[IBIS Ver]   4.1
[File Name]   rm57l843zwt.ibs
[File Rev]   1.0
[Date]   Mon Sep 1 2015 15:18:58
[Source]   Texas Instruments, Inc.
[Notes]   Revision History:
   1.0: initial release
   THE CONTENTS ARE SUBJECT TO CHANGE
   WITHOUT PRIOR NOTICE,IF NECESSARY.
[Disclaimer] Please be aware that in the absence of a written agreement
   Texas Instruments(TI) assumes no liability for:
   (1) The accuracy of the IBIS models provided to your company
   (2) The proper functioning of these Models in your design
   or for any resulting applications;or
   (3) Infringement of patents,copyrights or intellectual
   property rights resulting from your use of these models.
   TI provides IBIS Models as a service to our customers and
   therefore reserves the right to limit distribution of the
   Models.
[Copyright]   Property of Texas Instruments Incorporated.
   Unauthorised reproduction and/or distribution is strictly.
   prohibited.
   This product is protected under copyright law and trade
   secret law as an unpublished work.
   Created 2015,(C) Copyright 2015
   Texas Instruments Incorporated., All Rights Reserved.
   These commodities are under the U.S. Government
   distribution license control.As such,they are not to be
   re-exported without the prior approval of the
   U.S. Department of Commerce.
[Component]   rm57l843zwt
[Manufacturer]   Texas Instruments
[Package]
|variable   typ   min   max
R_pkg   167.768m   72.6527m   328.833m
L_pkg   2.60458nH   0.744426nH   6.40059nH
C_pkg   0.769905pF   0.48274pF   1.90756pF
[Pin] signal_name   model_name   R_pin   L_pin   C_pin
N19   AD1EVT/MII_RX_ER/RMII_RX_ER/NTZ1_1   BQ0210FS_PD_3X2_7LM_N19   180.1m   2.91nH   0.5019pF
T10   AD2EVT   BQ0210FS_PD_3X2_7LM_T10   191.2m   3.039nH  0.6641pF
B10   DCAN1RX   BQ0210FS_PU_3X2_7LM_B10   168.1m   2.756nH  0.712pF
A10   DCAN1TX   BQ0210FS_PU_3X2_7LM_A10   2190m   3.509nH  0.6666pF
H1   DCAN2RX   BQ0210FS_PU_3X2_7LM_H1   209.7m   3.041nH  0.5571pF
H2   DCAN2TX   BQ0210FS_PU_3X2_7LM_H2   161.2m   2.424nH  0.6686pF
M19   DCAN3RX   BQ0210FS_PU_3X2_7LM_M19   212.9m   3.153nH  0.5852pF
M18   DCAN3TX   BQ0210FS_PU_3X2_7LM_M18   195.7m   2.562nH  0.584pF
F17   DMM_CLK   BQ0210FS_PU_3X2_7LM_F17   159.7m   2.313nH  0.8981pF
L19   DMM_DATA[0]   BQ0210FS_PU_3X2_7LM_L19   211.2m   3.159nH  0.62pF
L18   DMM_DATA[1]   BQ0210FS_PU_3X2_7LM_L18   198.1m   2.749nH  0.6265pF
F16   DMM_NENA   BQ0210FS_PU_3X2_7LM_F16   1790m   2.494nH  1.017pF
J16   DMM_SYNC   BQ0210FS_PU_3X2_7LM_J16   153.5m   1.923nH  0.7789pF
A12   ECLK1   BQ0215FS_PD_3X2_V2_7LM_A12   227.3m   3.717nH  0.7204pF
D4   EMIF_ADDR[0]/N2HET2[1]   BQ0215FS_PD_3X2_7LM_D4   1070m   1.533nH  0.7807pF
C8   EMIF_ADDR[10]/RTP_DATA[9]   BQ0212FS_PD_3X2_7LM_C8   188.2m   2.407nH  0.6629pF
C9   EMIF_ADDR[11]/RTP_DATA[8]   BQ0212FS_PD_3X2_7LM_C9   202.5m   2.785nH  0.7576pF
C10   EMIF_ADDR[12]/RTP_DATA[6]   BQ0212FS_PD_3X2_7LM_C10   111.1m   1.862nH  0.7207pF
C11   EMIF_ADDR[13]/RTP_DATA[5]   BQ0212FS_PD_3X2_7LM_C11   142.7m   2.016nH  0.7216pF
C12   EMIF_ADDR[14]/RTP_DATA[4]   BQ0212FS_PD_3X2_7LM_C12   1920m   2.49nH   0.665pF
C13   EMIF_ADDR[15]/RTP_DATA[3]   BQ0212FS_PD_3X2_7LM_C13   148.4m   2.075nH  0.7037pF
D14   EMIF_ADDR[16]/RTP_DATA[2]   BQ0212FS_PD_3X2_7LM_D14   214.4m   2.798nH  0.7339pF
C14   EMIF_ADDR[17]/RTP_DATA[1]   BQ0212FS_PD_3X2_7LM_C14   133.3m   1.757nH  0.6447pF
D15   EMIF_ADDR[18]/RTP_DATA[0]   BQ0212FS_PD_3X2_7LM_D15   88.7m   1.066nH  0.6122pF
C15   EMIF_ADDR[19]/RTP_NENA   BQ0212FS_PU_3X2_7LM_C15   98.16m   1.386nH  0.6734pF
D5   EMIF_ADDR[1]/N2HET2[3]   BQ0215FS_PD_3X2_7LM_D5   155.7m   2.37nH   0.7927pF
C16   EMIF_ADDR[20]/RTP_NSYNC   BQ0212FS_PU_3X2_7LM_C16   126.9m   2.354nH  0.7879pF
C17   EMIF_ADDR[21]/RTP_CLK   BQ0212FS_PD_3X2_7LM_C17   179.7m   3.038nH  0.9204pF
C4   EMIF_ADDR[6]/RTP_DATA[13]/N2HET2[11]   BQ0215FS_PD_3X2_7LM_C4   217.2m   3.345nH  0.7595pF
C5   EMIF_ADDR[7]/RTP_DATA[12]/N2HET2[13]   BQ0215FS_PD_3X2_7LM_C5   209.2m   3.071nH  0.7332pF
C6   EMIF_ADDR[8]/RTP_DATA[11]/N2HET2[15]   BQ0215FS_PD_3X2_7LM_C6   151.8m   2.305nH  0.7583pF
C7   EMIF_ADDR[9]/RTP_DATA[10]   BQ0212FS_PD_3X2_7LM_C7   2130m   3.027nH  0.7353pF
D16   EMIF_BA[1]/N2HET2[5]   BQ0215FS_PD_3X2_7LM_D16   103.4m   1.556nH  0.6773pF
L3   EMIF_CKE   BQ0212FS_3X2_7LM_L3   188.4m   2.315nH  0.6502pF
R4   EMIF_NCAS/GIOB[3]   BQ0215FS_PD_3X2_7LM_R4   98.03m   1.629nH  0.901pF
N17   EMIF_NCS[0]/RTP_DATA[15]/N2HET2[7]   BQ0215FS_PD_3X2_7LM_N17   215.8m   2.667nH  0.6805pF
L17   EMIF_NCS[2]/GIOB[4]   BQ0215FS_PD_3X2_7LM_L17   1930m   2.377nH  0.6608pF
K17   EMIF_NCS[3]/RTP_DATA[14]/N2HET2[9]   BQ0215FS_PD_3X2_7LM_K17   140.2m   1.913nH  0.6591pF
M17   EMIF_NCS[4]/RTP_DATA[7]/GIOB[5]   BQ0215FS_PD_3X2_7LM_M17   141.2m   1.851nH  0.622pF
R3   EMIF_NRAS/GIOB[6]   BQ0215FS_PD_3X2_7LM_R3   169.2m   2.599nH  0.9236pF
P3   EMIF_NWAIT/GIOB[7]   BQ0210FS_PU_3X2_7LM_P3   225.8m   3.417nH  0.7552pF
D17   EMIF_NWE/EMIF_RNW   BQ0212FS_3X2_7LM_D17   248.5m   4.299nH  0.9019pF
D9   EPWM1A   BQ0212FS_3X2_7LM_D9   154.3m   2.317nH  0.7824pF
D10   EPWM1B   BQ0212FS_3X2_7LM_D10   157.6m   2.386nH  0.7576pF
R12   ETMDATA[0]   BQ0212FS_PD_3X2_7LM_R12   202.1m   3.095nH  1.034pF
E7   ETMDATA[10]/EMIF_ADDR[3]   BQ0212FS_PD_3X2_7LM_E7   155.1m   2.109nH  0.8648pF
E6   ETMDATA[11]/EMIF_ADDR[2]   BQ0212FS_PD_3X2_7LM_E6   152.7m   2.049nH  0.8297pF
E13   ETMDATA[12]/EMIF_BA[0]   BQ0212FS_PD_3X2_7LM_E13   150.6m   1.764nH  0.8299pF
E12   ETMDATA[13]/EMIF_NOE   BQ0212FS_PD_3X2_7LM_E12   84.46m   0.9329nH 0.7552pF
E11   ETMDATA[14]/EMIF_NDQM[1]   BQ0212FS_PD_3X2_7LM_E11   153.2m   2.043nH  0.8118pF
E10   ETMDATA[15]/EMIF_NDQM[0]   BQ0212FS_PD_3X2_7LM_E10   109.9m   1.609nH  0.8404pF
K15   ETMDATA[16]/EMIF_DATA[0]   BQ0212FS_PD_3X2_7LM_K15   159.5m   1.94nH   0.8165pF
L15   ETMDATA[17]/EMIF_DATA[1]   BQ0212FS_PD_3X2_7LM_L15   84.09m   0.8806nH 0.7489pF
M15   ETMDATA[18]/EMIF_DATA[2]   BQ0212FS_PD_3X2_7LM_M15   85.91m   0.9272nH 0.731pF
N15   ETMDATA[19]/EMIF_DATA[3]   BQ0212FS_PD_3X2_7LM_N15   161.4m   2.138nH  0.8751pF
R13   ETMDATA[1]   BQ0212FS_PD_3X2_7LM_R13   188.1m   3.032nH  0.8543pF
E5   ETMDATA[20]/EMIF_DATA[4]   BQ0212FS_PD_3X2_7LM_E5   80.68m   0.9128nH 0.7639pF
F5   ETMDATA[21]/EMIF_DATA[5]   BQ0212FS_PD_3X2_7LM_F5   72.65m   0.7444nH 0.7859pF
G5   ETMDATA[22]/EMIF_DATA[6]   BQ0212FS_PD_3X2_7LM_G5   72.98m   0.764nH  0.8191pF
K5   ETMDATA[23]/EMIF_DATA[7]   BQ0212FS_PD_3X2_7LM_K5   193.6m   3.113nH  0.8967pF
L5   ETMDATA[24]/EMIF_DATA[8]/N2HET2[24]   BQ0215FS_PD_3X2_7LM_L5   159.5m   2.044nH  0.8204pF
M5   ETMDATA[25]/EMIF_DATA[9]/N2HET2[25]   BQ0215FS_PD_3X2_7LM_M5   173.7m   2.268nH  0.9365pF
N5   ETMDATA[26]/EMIF_DATA[10]/N2HET2[26]   BQ0215FS_PD_3X2_7LM_N5   92.81m   1.339nH  0.8495pF
P5   ETMDATA[27]/EMIF_DATA[11]/N2HET2[27]   BQ0215FS_PD_3X2_7LM_P5   185.9m   2.57nH   1.034pF
R5   ETMDATA[28]/EMIF_DATA[12]/N2HET2[28]   BQ0215FS_PD_3X2_7LM_R5   1530m   1.982nH  0.785pF
R6   ETMDATA[29]/EMIF_DATA[13]/N2HET2[29]   BQ0215FS_PD_3X2_7LM_R6   74.23m   0.7853nH 0.778pF
J15   ETMDATA[2]   BQ0212FS_PD_3X2_7LM_J15   107.3m   1.449nH  0.8099pF
R7   ETMDATA[30]/EMIF_DATA[14]/N2HET2[30]   BQ0215FS_PD_3X2_7LM_R7   148.5m   1.714nH  0.7773pF
R8   ETMDATA[31]/EMIF_DATA[15]/N2HET2[31]   BQ0215FS_PD_3X2_7LM_R8   225.5m   3.11nH   0.8367pF
H15   ETMDATA[3]   BQ0212FS_PD_3X2_7LM_H15   101.3m   1.313nH  0.9263pF
G15   ETMDATA[4]   BQ0212FS_PD_3X2_7LM_G15   101.7m   1.315nH  0.9365pF
F15   ETMDATA[5]   BQ0212FS_PD_3X2_7LM_F15   176.6m   2.428nH  1.031pF
E15   ETMDATA[6]   BQ0212FS_PD_3X2_7LM_E15   88.42m   0.9896nH 0.7292pF
E14   ETMDATA[7]   BQ0212FS_PD_3X2_7LM_E14   111.4m   1.599nH  0.8526pF
E9   ETMDATA[8]/EMIF_ADDR[5]   BQ0212FS_PD_3X2_7LM_E9   98.29m   1.309nH  0.8713pF
E8   ETMDATA[9]/EMIF_ADDR[4]   BQ0212FS_PD_3X2_7LM_E8   123.3m   2.074nH  0.9081pF
R9   ETMTRACECLKIN/EXTCLKIN2/GIOA[5]   BQ0210FS_PU_3X2_7LM_R9   146.4m   1.723nH  0.8228pF
R10   ETMTRACECLKOUT/GIOA[6]   BQ0215FS_PD_3X2_7LM_R10   174.9m   2.651nH  0.8514pF
R11   ETMTRACECTL/GIOA[7]   BQ0215FS_PD_3X2_7LM_R11   165.4m   2.327nH  0.8792pF
A5   GIOA[0]   BQ0210FS_PD_3X2_7LM_A5   174.4m   3.024nH  0.6294pF
C2   GIOA[1]   BQ0210FS_PD_3X2_7LM_C2   147.5m   2.81nH   0.7829pF
C1   GIOA[2]/N2HET2[0]/EQEP2I   BQ0215FS_PD_3X2_7LM_C1   155.3m   3.055nH  0.8123pF
E1   GIOA[3]/N2HET2[2]   BQ0210FS_PD_3X2_7LM_E1   1920m   2.742nH  0.5404pF
A6   GIOA[4]   BQ0210FS_PD_3X2_7LM_A6   215.4m   3.36nH   0.6779pF
B5   GIOA[5]/EXTCLKIN/EPWM1A   BQ0215FS_PD_3X2_7LM_B5   284.7m   5.975nH  1.245pF
H3   GIOA[6]/N2HET2[4]/EPWM1B   BQ0215FS_PD_3X2_7LM_H3   138.7m   1.799nH  0.6061pF
M1   GIOA[7]/N2HET2[6]/EPWM2A   BQ0215FS_PD_3X2_7LM_M1   1780m   3.002nH  0.675pF
M2   GIOB[0]   BQ0210FS_PD_3X2_7LM_M2   188.9m   2.501nH  0.5986pF
K2   GIOB[1]   BQ0210FS_PD_3X2_7LM_K2   233.4m   3.564nH  0.693pF
F2   GIOB[2]/DCAN4TX   BQ0210FS_PD_3X2_7LM_F2   228.7m   3.418nH  0.6626pF
W10   GIOB[3]/DCAN4RX   BQ0210FS_PD_3X2_7LM_W10   221.6m   3.544nH  0.6783pF
G1   GIOB[4]   BQ0210FS_PD_3X2_7LM_G1   2090m   3.042nH  0.5395pF
G2   GIOB[5]   BQ0210FS_PD_3X2_7LM_G2   189.6m   2.519nH  0.543pF
J2   GIOB[6]/NERROR1   BQ0215FS_PD_3X2_7LM_J2   1930m   2.612nH  0.6214pF
F1   GIOB[7]/NERROR2/NTZ1_2   BQ0215FS_PD_3X2_7LM_F1   192.3m   2.707nH  0.5387pF
A7   LIN1RX   BQ0210FS_PU_3X2_7LM_A7   209.8m   3.283nH  0.6664pF
B7   LIN1TX   BQ0210FS_PU_3X2_7LM_B7   166.2m   2.66nH   0.7326pF
T9   MDCLK   BQ0212FS_3X2_7LM_T9   206.4m   2.691nH  0.7134pF
F4   MDIO   BQ0212FS_PD_3X2_7LM_F4   134.2m   1.553nH  0.7365pF
F18   MIBSPI1CLK   BQ0212FS_PU_3X2_V2_7LM_F18   163.9m   2.609nH  0.8532pF
R2   MIBSPI1NCS[0]/MIBSPI1SOMI[1]/ECAP6   BQ0215FS_PU_3X2_V2_7LM_R2   2040m   3.069nH  0.7035pF
F3   MIBSPI1NCS[1]/MII_COL/N2HET1[17]   BQ0215FS_PU_3X2_V2_7LM_F3   135.2m   1.767nH  0.7006pF
G3   MIBSPI1NCS[2]/MDIO/N2HET1[19]   BQ0215FS_PU_3X2_V2_7LM_G3   134.3m   1.738nH  0.6061pF
J3   MIBSPI1NCS[3]/N2HET1[21]/NTZ1_3   BQ0210FS_PU_3X2_V2_7LM_J3   141.8m   1.878nH  0.6604pF
U10   MIBSPI1NCS[4]   BQ0210FS_PU_3X2_V2_7LM_U10   210.9m   3.131nH  0.742pF
U9   MIBSPI1NCS[5]   BQ0210FS_PU_3X2_V2_7LM_U9   138.7m   1.953nH  0.7238pF
G19   MIBSPI1NENA/MII_RXD[2]/N2HET1[23]   BQ0215FS_PU_3X2_V2_7LM_G19   201.8m   3.617nH  0.8012pF
F19   MIBSPI1SIMO[0]   BQ0212FS_PU_3X2_V2_7LM_F19   188.7m   3.395nH  0.7797pF
G18   MIBSPI1SOMI[0]   BQ0212FS_PU_3X2_V2_7LM_G18   240.1m   3.78nH   0.7331pF
V9   MIBSPI3CLK/AD1EXT_SEL[1]/EQEP1A   BQ0215FS_PU_3X2_V2_7LM_V9   199.7m   2.886nH  0.6979pF
V10   MIBSPI3NCS[0]/AD2EVT/EQEP1I   BQ0215FS_PU_3X2_V2_7LM_V10   158.2m   2.499nH  0.7082pF
V5   MIBSPI3NCS[1]/MDCLK/N2HET1[25]   BQ0215FS_PU_3X2_V2_7LM_V5   106.2m   1.818nH  0.6775pF
B2   MIBSPI3NCS[2]/I2C1_SDA/N2HET1[27]   BQ0210FS_PU_3X2_V2_7LM_B2   139.4m   2.787nH  0.802pF
C3   MIBSPI3NCS[3]/I2C1_SCL/N2HET1[29]   BQ0210FS_PU_3X2_V2_7LM_C3   133.3m   2.406nH  0.7799pF
W9   MIBSPI3NENA/MIBSPI3NCS[5]/N2HET1[31]   BQ0210FS_PU_3X2_V2_7LM_W9   1860m   3.246nH  0.7361pF
W8   MIBSPI3SIMO/AD1EXT_SEL[0]/ECAP3   BQ0215FS_PU_3X2_V2_7LM_W8   222.3m   3.401nH  0.6785pF
V8   MIBSPI3SOMI/AD1EXT_ENA/ECAP2   BQ0215FS_PU_3X2_V2_7LM_V8   196.3m   2.655nH  0.6375pF
H19   MIBSPI5CLK/DMM_DATA[4]/MII_TXEN   BQ0215FS_PU_3X2_V2_7LM_H19   215.9m   3.255nH  0.6747pF
E19   MIBSPI5NCS[0]/DMM_DATA[5]/EPWM4A   BQ0215FS_PU_3X2_V2_7LM_E19   195.1m   3.655nH  0.7715pF
B6   MIBSPI5NCS[1]/DMM_DATA[6]   BQ0210FS_PU_3X2_V2_7LM_B6   163.8m   2.656nH  0.7413pF
W6   MIBSPI5NCS[2]/DMM_DATA[2]   BQ0210FS_PU_3X2_V2_7LM_W6   226.5m   3.636nH  0.6405pF
T12   MIBSPI5NCS[3]/DMM_DATA[3]   BQ0210FS_PU_3X2_V2_7LM_T12   243.7m   3.684nH  0.8617pF
H18   MIBSPI5NENA/DMM_DATA[7]/MII_RXD[3]   BQ0215FS_PU_3X2_V2_7LM_H18   175.1m   2.788nH  0.7475pF
J19   MIBSPI5SIMO[0]/DMM_DATA[8]/MII_TXD[1]   BQ0215FS_PU_3X2_V2_7LM_J19   213.8m   3.285nH  0.6432pF
E16   MIBSPI5SIMO[1]/DMM_DATA[9]   BQ0215FS_PU_3X2_V2_7LM_E16   162.6m   2.366nH  0.9935pF
H17   MIBSPI5SIMO[2]/DMM_DATA[10]   BQ0215FS_PU_3X2_V2_7LM_H17   212.2m   2.843nH  0.7812pF
G17   MIBSPI5SIMO[3]/DMM_DATA[11]/I2C2_SDA   BQ0215FS_PU_3X2_V2_7LM_G17   1260m   2.223nH  0.877pF
J18   MIBSPI5SOMI[0]/DMM_DATA[12]/MII_TXD[0]  BQ0215FS_PU_3X2_V2_7LM_J18   210.6m   3.033nH  0.6889pF
E17   MIBSPI5SOMI[1]/DMM_DATA[13]   BQ0215FS_PU_3X2_V2_7LM_E17   216.2m   3.07nH   0.9498pF
H16   MIBSPI5SOMI[2]/DMM_DATA[14]   BQ0215FS_PU_3X2_V2_7LM_H16   149.5m   1.898nH  0.7973pF
G16   MIBSPI5SOMI[3]/DMM_DATA[15]/I2C2_SCL   BQ0215FS_PU_3X2_V2_7LM_G16   151.4m   2.031nH  0.8541pF
W4   MII_COL   IQ0088FS_PU_3X2_7LM_W4   187.5m   4.177nH  1.059pF
V4   MII_CRS   IQ0088FS_PD_3X2_7LM_V4   1620m   3.281nH  1.03pF
T4   MII_RXCLK   BQ0212FS_PD_3X2_7LM_T4   94.56m   1.282nH  0.7619pF
U4   MII_RXD[0]   IQ0088FS_PD_3X2_7LM_U4   106.7m   1.722nH  0.8846pF
T3   MII_RXD[1]   IQ0088FS_PD_3X2_7LM_T3   1680m   2.789nH  0.9027pF
U3   MII_RXD[2]   IQ0088FS_PD_3X2_7LM_U3   114.9m   2.194nH  0.8787pF
V3   MII_RXD[3]   IQ0088FS_PD_3X2_7LM_V3   185.4m   3.222nH  0.9958pF
U6   MII_RX_DV   IQ0088FS_PD_3X2_7LM_U6   139.3m   1.843nH  0.6451pF
U5   MII_RX_ER   IQ0088FS_PD_3X2_7LM_U5   85.96m   1.253nH  0.6256pF
U8   MII_TXD[0]   BQ0212FS_3X2_7LM_U8   133.8m   1.674nH  0.6851pF
R1   MII_TXD[1]   BQ0212FS_3X2_7LM_R1   219.5m   3.473nH  0.6574pF
T2   MII_TXD[2]   BQ0212FS_3X2_7LM_T2   165.1m   2.802nH  0.7483pF
G4   MII_TXD[3]   BQ0212FS_3X2_7LM_G4   1350m   1.589nH  0.6504pF
E4   MII_TXEN   BQ0212FS_3X2_7LM_E4   1500m   1.981nH  0.7545pF
U7   MII_TX_CLK   BQ0212FS_PD_3X2_7LM_U7   138.7m   1.81nH   0.6528pF
K18   N2HET1[0]/MIBSPI4CLK/EPWM2B   BQ0215FS_PD_3X2_V2_7LM_K18   194.9m   2.618nH  0.6421pF
D19   N2HET1[10]/MIBSPI4NCS[4]/MII_TX_CLK   BQ0215FS_PD_3X2_V2_7LM_D19   238.1m   3.959nH  0.783pF
E3   N2HET1[11]/MIBSPI3NCS[4]/N2HET2[18]   BQ0210FS_PD_3X2_V2_7LM_E3   230.1m   3.559nH  0.6823pF
B4   N2HET1[12]/MIBSPI4NCS[5]/MII_CRS   BQ0216FS_PD_3X2_7LM_B4   171.4m   2.841nH  0.7273pF
N2   N2HET1[13]/SCI3TX/N2HET2[20]/EPWM5B   BQ0215FS_PD_3X2_7LM_N2   228.7m   3.496nH  0.6574pF
A11   N2HET1[14]   BQ0210FS_PD_3X2_7LM_A11   188.6m   3.406nH  0.7399pF
N1   N2HET1[15]/MIBSPI1NCS[4]/N2HET2[22]   BQ0215FS_PD_3X2_V2_7LM_N1   175.4m   3.029nH  0.5725pF
A4   N2HET1[16]/EPWM1SYNCI/EPWM1SYNCO   BQ0210FS_PD_3X2_7LM_A4   213.8m   3.403nH  0.6157pF
A13   N2HET1[17]/EMIF_NOE/SCI4RX   BQ0215FS_PD_3X2_7LM_A13   192.4m   3.468nH  0.7729pF
J1   N2HET1[18]/EMIF_RNW/EPWM6A   BQ0215FS_PD_3X2_7LM_J1   211.3m   3.101nH  0.6108pF
B13   N2HET1[19]/EMIF_NDQM[0]/SCI4TX   BQ0215FS_PD_3X2_7LM_B13   203.8m   2.896nH  0.6717pF
V2   N2HET1[1]/MIBSPI4NENA/N2HET2[8]/EQEP2A  BQ0215FS_PD_3X2_V2_7LM_V2   243.7m   4.212nH  0.8788pF
P2   N2HET1[20]/EMIF_NDQM[1]/EPWM6B   BQ0215FS_PD_3X2_7LM_P2   197.3m   3.478nH  0.7551pF
H4   N2HET1[21]/EMIF_NDQM[2]   BQ0215FS_PD_3X2_7LM_H4   80.72m   1.038nH  0.6588pF
B3   N2HET1[22]/EMIF_NDQM[3]   BQ0215FS_PD_3X2_7LM_B3   238.4m   3.878nH  0.74pF
J4   N2HET1[23]/EMIF_BA[0]   BQ0215FS_PD_3X2_7LM_J4   77.83m   1.03nH   0.6535pF
P1   N2HET1[24]/MIBSPI1NCS[5]/MII_RXD[0]   BQ0210FS_PD_3X2_V2_7LM_P1   217.2m   3.308nH  0.5921pF
M3   N2HET1[25]   BQ0210FS_PD_3X2_7LM_M3   194.9m   2.47nH   0.6778pF
A14   N2HET1[26]/MII_RXD[1]/RMII_RXD[1]   BQ0210FS_PD_3X2_7LM_A14   195.1m   3.44nH   0.7296pF
A9   N2HET1[27]   BQ0210FS_PD_3X2_7LM_A9   2220m   3.586nH  0.7024pF
K19   N2HET1[28]/MII_RXCLK/RMII_REFCLK   BQ0215FS_PD_3X2_7LM_K19   178.6m   2.973nH  0.6837pF
A3   N2HET1[29]   BQ0210FS_PD_3X2_7LM_A3   177.8m   3.069nH  0.7881pF
W5   N2HET1[2]/MIBSPI4SIMO/EPWM3A   BQ0215FS_PD_3X2_V2_7LM_W5   131.6m   2.509nH  0.7814pF
B11   N2HET1[30]/MII_RX_DV/EQEP2S   BQ0215FS_PD_3X2_7LM_B11   199.7m   2.90nH   0.6704pF
J17   N2HET1[31]   BQ0210FS_PD_3X2_7LM_J17   182.8m   2.671nH  0.768pF
U1   N2HET1[3]/MIBSPI4NCS[0]/N2HET2[10]   BQ0210FS_PD_3X2_V2_7LM_U1   232.4m   3.951nH  0.7369pF
B12   N2HET1[4]/MIBSPI4NCS[1]/EPWM4B   BQ0215FS_PD_3X2_V2_7LM_B12   169.8m   2.767nH  0.7311pF
V6   N2HET1[5]/MIBSPI4SOMI/N2HET2[12]   BQ0215FS_PD_3X2_V2_7LM_V6   184.1m   2.418nH  0.4827pF
W3   N2HET1[6]/SCI3RX/EPWM5A   BQ0215FS_PD_3X2_7LM_W3   250.6m   4.817nH  1.046pF
T1   N2HET1[7]/MIBSPI4NCS[2]/N2HET2[14]   BQ0215FS_PD_3X2_V2_7LM_T1   224.8m   3.67nH   0.6807pF
E18   N2HET1[8]/MIBSPI1SIMO[1]/MII_TXD[3]   BQ0215FS_PD_3X2_V2_7LM_E18   2550m   4.358nH  0.8333pF
V7   N2HET1[9]/MIBSPI4NCS[3]/N2HET2[16]   BQ0215FS_PD_3X2_V2_7LM_V7   192.6m   2.597nH  0.6235pF
D6   N2HET2[0]   BQ0210FS_PD_3X2_7LM_D6   206.5m   2.777nH  0.7604pF
M16   N2HET2[10]   BQ0210FS_PD_3X2_7LM_M16   139.1m   1.655nH  0.6675pF
N16   N2HET2[11]   BQ0210FS_PD_3X2_7LM_N16   162.6m   2.153nH  0.7516pF
D3   N2HET2[12]/MIBSPI2NENA/MIBSPI2NCS[1]   BQ0210FS_PD_3X2_V2_7LM_D3   89.21m   1.356nH  0.6802pF
D2   N2HET2[13]/MIBSPI2SOMI   BQ0215FS_PD_3X2_V2_7LM_D2   103.4m   1.818nH  0.6291pF
D1   N2HET2[14]/MIBSPI2SIMO   BQ0215FS_PD_3X2_V2_7LM_D1   124.7m   2.391nH  0.671pF
K4   N2HET2[15]   BQ0210FS_PD_3X2_7LM_K4   143.4m   1.768nH  0.705pF
L4   N2HET2[16]   BQ0210FS_PD_3X2_7LM_L4   75.57m   0.9412nH 0.6801pF
M4   N2HET2[17]   BQ0210FS_PD_3X2_7LM_M4   141.6m   1.746nH  0.7459pF
N4   N2HET2[18]   BQ0210FS_PD_3X2_7LM_N4   1490m   2.004nH  0.7947pF
P4   N2HET2[19]/LIN2RX   BQ0210FS_PD_3X2_7LM_P4   148.1m   1.945nH  0.8194pF
D8   N2HET2[1]/N2HET1_NDIS   BQ0210FS_PD_3X2_7LM_D8   133.3m   1.583nH  0.7411pF
T5   N2HET2[20]/LIN2TX   BQ0210FS_PD_3X2_7LM_T5   76.75m   0.981nH  0.6626pF
T6   N2HET2[21]   BQ0210FS_PD_3X2_7LM_T6   129.9m   1.501nH  0.6862pF
T7   N2HET2[22]   BQ0210FS_PD_3X2_7LM_T7   201.8m   2.486nH  0.7263pF
T8   N2HET2[23]   BQ0210FS_PD_3X2_7LM_T8   129.9m   1.514nH  0.6737pF
D7   N2HET2[2]/N2HET2_NDIS   BQ0210FS_PD_3X2_7LM_D7   209.5m   2.805nH  0.7737pF
E2   N2HET2[3]/MIBSPI2CLK   BQ0215FS_PD_3X2_V2_7LM_E2   158.4m   2.411nH  0.6091pF
D13   N2HET2[4]   BQ0210FS_PD_3X2_7LM_D13   208.2m   2.68nH   0.7825pF
D12   N2HET2[5]   BQ0210FS_PD_3X2_7LM_D12   140.1m   1.755nH  0.7326pF
D11   N2HET2[6]   BQ0210FS_PD_3X2_7LM_D11   101.9m   1.511nH  0.7759pF
N3   N2HET2[7]/MIBSPI2NCS[0]   BQ0210FS_PD_3X2_V2_7LM_N3   150.2m   2.212nH  0.7463pF
K16   N2HET2[8]   BQ0210FS_PD_3X2_7LM_K16   2130m   2.65nH   0.7726pF
L16   N2HET2[9]   BQ0210FS_PD_3X2_7LM_L16   138.3m   1.599nH  0.7153pF
B14   NERROR   BQ0212FS_PD_3X2_7LM_B14   212.7m   3.079nH  0.6773pF
W7   NPORRST   IQ0087FS_3X2_7LM_W7   220.5m   3.413nH  0.6666pF
B17   NRST   BQ0414FS_DL_3X2_7LM_B17   2620m   4.571nH  0.9293pF
D18   NTRST   IQ0087FS_3X2_7LM_D18   195.7m   3.535nH  0.9233pF
A16   RTCK   BQ0212FS_3X2_7LM_A16   162.5m   3.459nH  0.9192pF
B18   TCK   IQ0079FS_PD_3X2_7LM_B18   244.6m   4.88nH   1.012pF
A17   TDI   BQ0192FS_PU_3X2_7LM_A17   234.9m   4.677nH  1.047pF
C18   TDO   BQ0192FS_PD_3X2_7LM_C18   245.6m   4.219nH  0.8864pF
U2   TEST   BQ0213FS_PD_3X2_7LM_U2   181.6m   3.211nH  0.8308pF
C19   TMS   BQ0192FS_PU_3X2_7LM_C19   246.7m   4.332nH  0.8139pF
[Model Selector]   BQ0192FS_PD_3X2_7LM_C18
BQ0192FS_PD_3X2_7LM_PZ_3P3  Cell operated at 3
|BQ0192FS_PD_3X2_7LM_PZ_3P3; PUPD_OFF
BQ0192FS_PD_3X2_7LM_PU_3P3  Cell operated at 3
|BQ0192FS_PD_3X2_7LM_PU_3P3; PULLUP_ON
BQ0192FS_PD_3X2_7LM_PD_3P3  Cell operated at 3
|BQ0192FS_PD_3X2_7LM_PD_3P3; PULLDOWN_ON
[Model Selector]   BQ0192FS_PU_3X2_7LM_A17
BQ0192FS_PU_3X2_7LM_PZ_3P3  Cell operated at 3
|BQ0192FS_PU_3X2_7LM_PZ_3P3; PUPD_OFF
BQ0192FS_PU_3X2_7LM_PU_3P3  Cell operated at 3
|BQ0192FS_PU_3X2_7LM_PU_3P3; PULLUP_ON
BQ0192FS_PU_3X2_7LM_PD_3P3  Cell operated at 3
|BQ0192FS_PU_3X2_7LM_PD_3P3; PULLDOWN_ON
[Model Selector]   BQ0192FS_PU_3X2_7LM_C19
BQ0192FS_PU_3X2_7LM_PZ_3P3  Cell operated at 3
|BQ0192FS_PU_3X2_7LM_PZ_3P3; PUPD_OFF
BQ0192FS_PU_3X2_7LM_PU_3P3  Cell operated at 3
|BQ0192FS_PU_3X2_7LM_PU_3P3; PULLUP_ON
BQ0192FS_PU_3X2_7LM_PD_3P3  Cell operated at 3
|BQ0192FS_PU_3X2_7LM_PD_3P3; PULLDOWN_ON
[Model Selector]   BQ0210FS_PD_3X2_7LM_A11
BQ0210FS_PD_3X2_7LM_PZ_3P3  Cell operated at 3
|BQ0210FS_PD_3X2_7LM_PZ_3P3; PUPD_OFF
BQ0210FS_PD_3X2_7LM_PU_3P3  Cell operated at 3
|BQ0210FS_PD_3X2_7LM_PU_3P3; PULLUP_ON
BQ0210FS_PD_3X2_7LM_PD_3P3  Cell operated at 3
|BQ0210FS_PD_3X2_7LM_PD_3P3; PULLDOWN_ON
[Model Selector]   BQ0210FS_PD_3X2_7LM_A14
BQ0210FS_PD_3X2_7LM_PZ_3P3  Cell operated at 3
|BQ0210FS_PD_3X2_7LM_PZ_3P3; PUPD_OFF
BQ0210FS_PD_3X2_7LM_PU_3P3  Cell operated at 3
|BQ0210FS_PD_3X2_7LM_PU_3P3; PULLUP_ON
BQ0210FS_PD_3X2_7LM_PD_3P3  Cell operated at 3
|BQ0210FS_PD_3X2_7LM_PD_3P3; PULLDOWN_ON
[Model Selector]   BQ0210FS_PD_3X2_7LM_A3
BQ0210FS_PD_3X2_7LM_PZ_3P3  Cell operated at 3
|BQ0210FS_PD_3X2_7LM_PZ_3P3; PUPD_OFF
BQ0210FS_PD_3X2_7LM_PU_3P3  Cell operated at 3
|BQ0210FS_PD_3X2_7LM_PU_3P3; PULLUP_ON
BQ0210FS_PD_3X2_7LM_PD_3P3  Cell operated at 3
|BQ0210FS_PD_3X2_7LM_PD_3P3; PULLDOWN_ON
[Model Selector]   BQ0210FS_PD_3X2_7LM_A4
BQ0210FS_PD_3X2_7LM_PZ_3P3  Cell operated at 3
|BQ0210FS_PD_3X2_7LM_PZ_3P3; PUPD_OFF
BQ0210FS_PD_3X2_7LM_PU_3P3  Cell operated at 3
|BQ0210FS_PD_3X2_7LM_PU_3P3; PULLUP_ON
BQ0210FS_PD_3X2_7LM_PD_3P3  Cell operated at 3
|BQ0210FS_PD_3X2_7LM_PD_3P3; PULLDOWN_ON
[Model Selector]   BQ0210FS_PD_3X2_7LM_A5
BQ0210FS_PD_3X2_7LM_PZ_3P3  Cell operated at 3
|BQ0210FS_PD_3X2_7LM_PZ_3P3; PUPD_OFF
BQ0210FS_PD_3X2_7LM_PU_3P3  Cell operated at 3
|BQ0210FS_PD_3X2_7LM_PU_3P3; PULLUP_ON
BQ0210FS_PD_3X2_7LM_PD_3P3  Cell operated at 3
|BQ0210FS_PD_3X2_7LM_PD_3P3; PULLDOWN_ON
[Model Selector]   BQ0210FS_PD_3X2_7LM_A6
BQ0210FS_PD_3X2_7LM_PZ_3P3  Cell operated at 3
|BQ0210FS_PD_3X2_7LM_PZ_3P3; PUPD_OFF
BQ0210FS_PD_3X2_7LM_PU_3P3  Cell operated at 3
|BQ0210FS_PD_3X2_7LM_PU_3P3; PULLUP_ON
BQ0210FS_PD_3X2_7LM_PD_3P3  Cell operated at 3
|BQ0210FS_PD_3X2_7LM_PD_3P3; PULLDOWN_ON
[Model Selector]   BQ0210FS_PD_3X2_7LM_A9
BQ0210FS_PD_3X2_7LM_PZ_3P3  Cell operated at 3
|BQ0210FS_PD_3X2_7LM_PZ_3P3; PUPD_OFF
BQ0210FS_PD_3X2_7LM_PU_3P3  Cell operated at 3
|BQ0210FS_PD_3X2_7LM_PU_3P3; PULLUP_ON
BQ0210FS_PD_3X2_7LM_PD_3P3  Cell operated at 3
|BQ0210FS_PD_3X2_7LM_PD_3P3; PULLDOWN_ON
[Model Selector]   BQ0210FS_PD_3X2_7LM_C2
BQ0210FS_PD_3X2_7LM_PZ_3P3  Cell operated at 3
|BQ0210FS_PD_3X2_7LM_PZ_3P3; PUPD_OFF
BQ0210FS_PD_3X2_7LM_PU_3P3  Cell operated at 3
|BQ0210FS_PD_3X2_7LM_PU_3P3; PULLUP_ON
BQ0210FS_PD_3X2_7LM_PD_3P3  Cell operated at 3
|BQ0210FS_PD_3X2_7LM_PD_3P3; PULLDOWN_ON
[Model Selector]   BQ0210FS_PD_3X2_7LM_D11
BQ0210FS_PD_3X2_7LM_PZ_3P3  Cell operated at 3
|BQ0210FS_PD_3X2_7LM_PZ_3P3; PUPD_OFF
BQ0210FS_PD_3X2_7LM_PU_3P3  Cell operated at 3
|BQ0210FS_PD_3X2_7LM_PU_3P3; PULLUP_ON
BQ0210FS_PD_3X2_7LM_PD_3P3  Cell operated at 3
|BQ0210FS_PD_3X2_7LM_PD_3P3; PULLDOWN_ON
[Model Selector]   BQ0210FS_PD_3X2_7LM_D12
BQ0210FS_PD_3X2_7LM_PZ_3P3  Cell operated at 3
|BQ0210FS_PD_3X2_7LM_PZ_3P3; PUPD_OFF
BQ0210FS_PD_3X2_7LM_PU_3P3  Cell operated at 3
|BQ0210FS_PD_3X2_7LM_PU_3P3; PULLUP_ON
BQ0210FS_PD_3X2_7LM_PD_3P3  Cell operated at 3
|BQ0210FS_PD_3X2_7LM_PD_3P3; PULLDOWN_ON
[Model Selector]   BQ0210FS_PD_3X2_7LM_D13
BQ0210FS_PD_3X2_7LM_PZ_3P3  Cell operated at 3
|BQ0210FS_PD_3X2_7LM_PZ_3P3; PUPD_OFF
BQ0210FS_PD_3X2_7LM_PU_3P3  Cell operated at 3
|BQ0210FS_PD_3X2_7LM_PU_3P3; PULLUP_ON
BQ0210FS_PD_3X2_7LM_PD_3P3  Cell operated at 3
|BQ0210FS_PD_3X2_7LM_PD_3P3; PULLDOWN_ON
[Model Selector]   BQ0210FS_PD_3X2_7LM_D6
BQ0210FS_PD_3X2_7LM_PZ_3P3  Cell operated at 3
|BQ0210FS_PD_3X2_7LM_PZ_3P3; PUPD_OFF
BQ0210FS_PD_3X2_7LM_PU_3P3  Cell operated at 3
|BQ0210FS_PD_3X2_7LM_PU_3P3; PULLUP_ON
BQ0210FS_PD_3X2_7LM_PD_3P3  Cell operated at 3
|BQ0210FS_PD_3X2_7LM_PD_3P3; PULLDOWN_ON
[Model Selector]   BQ0210FS_PD_3X2_7LM_D7
BQ0210FS_PD_3X2_7LM_PZ_3P3  Cell operated at 3
|BQ0210FS_PD_3X2_7LM_PZ_3P3; PUPD_OFF
BQ0210FS_PD_3X2_7LM_PU_3P3  Cell operated at 3
|BQ0210FS_PD_3X2_7LM_PU_3P3; PULLUP_ON
BQ0210FS_PD_3X2_7LM_PD_3P3  Cell operated at 3
|BQ0210FS_PD_3X2_7LM_PD_3P3; PULLDOWN_ON
[Model Selector]   BQ0210FS_PD_3X2_7LM_D8
BQ0210FS_PD_3X2_7LM_PZ_3P3  Cell operated at 3
|BQ0210FS_PD_3X2_7LM_PZ_3P3; PUPD_OFF
BQ0210FS_PD_3X2_7LM_PU_3P3  Cell operated at 3
|BQ0210FS_PD_3X2_7LM_PU_3P3; PULLUP_ON
BQ0210FS_PD_3X2_7LM_PD_3P3  Cell operated at 3
|BQ0210FS_PD_3X2_7LM_PD_3P3; PULLDOWN_ON
[Model Selector]   BQ0210FS_PD_3X2_7LM_E1
BQ0210FS_PD_3X2_7LM_PZ_3P3  Cell operated at 3
|BQ0210FS_PD_3X2_7LM_PZ_3P3; PUPD_OFF
BQ0210FS_PD_3X2_7LM_PU_3P3  Cell operated at 3
|BQ0210FS_PD_3X2_7LM_PU_3P3; PULLUP_ON
BQ0210FS_PD_3X2_7LM_PD_3P3  Cell operated at 3
|BQ0210FS_PD_3X2_7LM_PD_3P3; PULLDOWN_ON
[Model Selector]   BQ0210FS_PD_3X2_7LM_F2
BQ0210FS_PD_3X2_7LM_PZ_3P3  Cell operated at 3
|BQ0210FS_PD_3X2_7LM_PZ_3P3; PUPD_OFF
BQ0210FS_PD_3X2_7LM_PU_3P3  Cell operated at 3
|BQ0210FS_PD_3X2_7LM_PU_3P3; PULLUP_ON
BQ0210FS_PD_3X2_7LM_PD_3P3  Cell operated at 3
|BQ0210FS_PD_3X2_7LM_PD_3P3; PULLDOWN_ON
[Model Selector]   BQ0210FS_PD_3X2_7LM_G1
BQ0210FS_PD_3X2_7LM_PZ_3P3  Cell operated at 3
|BQ0210FS_PD_3X2_7LM_PZ_3P3; PUPD_OFF
BQ0210FS_PD_3X2_7LM_PU_3P3  Cell operated at 3
|BQ0210FS_PD_3X2_7LM_PU_3P3; PULLUP_ON
BQ0210FS_PD_3X2_7LM_PD_3P3  Cell operated at 3
|BQ0210FS_PD_3X2_7LM_PD_3P3; PULLDOWN_ON
[Model Selector]   BQ0210FS_PD_3X2_7LM_G2
BQ0210FS_PD_3X2_7LM_PZ_3P3  Cell operated at 3
|BQ0210FS_PD_3X2_7LM_PZ_3P3; PUPD_OFF
BQ0210FS_PD_3X2_7LM_PU_3P3  Cell operated at 3
|BQ0210FS_PD_3X2_7LM_PU_3P3; PULLUP_ON
BQ0210FS_PD_3X2_7LM_PD_3P3  Cell operated at 3
|BQ0210FS_PD_3X2_7LM_PD_3P3; PULLDOWN_ON
[Model Selector]   BQ0210FS_PD_3X2_7LM_J17
BQ0210FS_PD_3X2_7LM_PZ_3P3  Cell operated at 3
|BQ0210FS_PD_3X2_7LM_PZ_3P3; PUPD_OFF
BQ0210FS_PD_3X2_7LM_PU_3P3  Cell operated at 3
|BQ0210FS_PD_3X2_7LM_PU_3P3; PULLUP_ON
BQ0210FS_PD_3X2_7LM_PD_3P3  Cell operated at 3
|BQ0210FS_PD_3X2_7LM_PD_3P3; PULLDOWN_ON
[Model Selector]   BQ0210FS_PD_3X2_7LM_K16
BQ0210FS_PD_3X2_7LM_PZ_3P3  Cell operated at 3
|BQ0210FS_PD_3X2_7LM_PZ_3P3; PUPD_OFF
BQ0210FS_PD_3X2_7LM_PU_3P3  Cell operated at 3
|BQ0210FS_PD_3X2_7LM_PU_3P3; PULLUP_ON
BQ0210FS_PD_3X2_7LM_PD_3P3  Cell operated at 3
|BQ0210FS_PD_3X2_7LM_PD_3P3; PULLDOWN_ON
[Model Selector]   BQ0210FS_PD_3X2_7LM_K2
BQ0210FS_PD_3X2_7LM_PZ_3P3  Cell operated at 3
|BQ0210FS_PD_3X2_7LM_PZ_3P3; PUPD_OFF
BQ0210FS_PD_3X2_7LM_PU_3P3  Cell operated at 3
|BQ0210FS_PD_3X2_7LM_PU_3P3; PULLUP_ON
BQ0210FS_PD_3X2_7LM_PD_3P3  Cell operated at 3
|BQ0210FS_PD_3X2_7LM_PD_3P3; PULLDOWN_ON
[Model Selector]   BQ0210FS_PD_3X2_7LM_K4
BQ0210FS_PD_3X2_7LM_PZ_3P3  Cell operated at 3
|BQ0210FS_PD_3X2_7LM_PZ_3P3; PUPD_OFF
BQ0210FS_PD_3X2_7LM_PU_3P3  Cell operated at 3
|BQ0210FS_PD_3X2_7LM_PU_3P3; PULLUP_ON
BQ0210FS_PD_3X2_7LM_PD_3P3  Cell operated at 3
|BQ0210FS_PD_3X2_7LM_PD_3P3; PULLDOWN_ON
[Model Selector]   BQ0210FS_PD_3X2_7LM_L16
BQ0210FS_PD_3X2_7LM_PZ_3P3  Cell operated at 3
|BQ0210FS_PD_3X2_7LM_PZ_3P3; PUPD_OFF
BQ0210FS_PD_3X2_7LM_PU_3P3  Cell operated at 3
|BQ0210FS_PD_3X2_7LM_PU_3P3; PULLUP_ON
BQ0210FS_PD_3X2_7LM_PD_3P3  Cell operated at 3
|BQ0210FS_PD_3X2_7LM_PD_3P3; PULLDOWN_ON
[Model Selector]   BQ0210FS_PD_3X2_7LM_L4
BQ0210FS_PD_3X2_7LM_PZ_3P3  Cell operated at 3
|BQ0210FS_PD_3X2_7LM_PZ_3P3; PUPD_OFF
BQ0210FS_PD_3X2_7LM_PU_3P3  Cell operated at 3
|BQ0210FS_PD_3X2_7LM_PU_3P3; PULLUP_ON
BQ0210FS_PD_3X2_7LM_PD_3P3  Cell operated at 3
|BQ0210FS_PD_3X2_7LM_PD_3P3; PULLDOWN_ON
[Model Selector]   BQ0210FS_PD_3X2_7LM_M16
BQ0210FS_PD_3X2_7LM_PZ_3P3  Cell operated at 3
|BQ0210FS_PD_3X2_7LM_PZ_3P3; PUPD_OFF
BQ0210FS_PD_3X2_7LM_PU_3P3  Cell operated at 3
|BQ0210FS_PD_3X2_7LM_PU_3P3; PULLUP_ON
BQ0210FS_PD_3X2_7LM_PD_3P3  Cell operated at 3
|BQ0210FS_PD_3X2_7LM_PD_3P3; PULLDOWN_ON
[Model Selector]   BQ0210FS_PD_3X2_7LM_M2
BQ0210FS_PD_3X2_7LM_PZ_3P3  Cell operated at 3
|BQ0210FS_PD_3X2_7LM_PZ_3P3; PUPD_OFF
BQ0210FS_PD_3X2_7LM_PU_3P3  Cell operated at 3
|BQ0210FS_PD_3X2_7LM_PU_3P3; PULLUP_ON
BQ0210FS_PD_3X2_7LM_PD_3P3  Cell operated at 3
|BQ0210FS_PD_3X2_7LM_PD_3P3; PULLDOWN_ON
[Model Selector]   BQ0210FS_PD_3X2_7LM_M3
BQ0210FS_PD_3X2_7LM_PZ_3P3  Cell operated at 3
|BQ0210FS_PD_3X2_7LM_PZ_3P3; PUPD_OFF
BQ0210FS_PD_3X2_7LM_PU_3P3  Cell operated at 3
|BQ0210FS_PD_3X2_7LM_PU_3P3; PULLUP_ON
BQ0210FS_PD_3X2_7LM_PD_3P3  Cell operated at 3
|BQ0210FS_PD_3X2_7LM_PD_3P3; PULLDOWN_ON
[Model Selector]   BQ0210FS_PD_3X2_7LM_M4
BQ0210FS_PD_3X2_7LM_PZ_3P3  Cell operated at 3
|BQ0210FS_PD_3X2_7LM_PZ_3P3; PUPD_OFF
BQ0210FS_PD_3X2_7LM_PU_3P3  Cell operated at 3
|BQ0210FS_PD_3X2_7LM_PU_3P3; PULLUP_ON
BQ0210FS_PD_3X2_7LM_PD_3P3  Cell operated at 3
|BQ0210FS_PD_3X2_7LM_PD_3P3; PULLDOWN_ON
[Model Selector]   BQ0210FS_PD_3X2_7LM_N16
BQ0210FS_PD_3X2_7LM_PZ_3P3  Cell operated at 3
|BQ0210FS_PD_3X2_7LM_PZ_3P3; PUPD_OFF
BQ0210FS_PD_3X2_7LM_PU_3P3  Cell operated at 3
|BQ0210FS_PD_3X2_7LM_PU_3P3; PULLUP_ON
BQ0210FS_PD_3X2_7LM_PD_3P3  Cell operated at 3
|BQ0210FS_PD_3X2_7LM_PD_3P3; PULLDOWN_ON
[Model Selector]   BQ0210FS_PD_3X2_7LM_N19
BQ0210FS_PD_3X2_7LM_PZ_3P3  Cell operated at 3
|BQ0210FS_PD_3X2_7LM_PZ_3P3; PUPD_OFF
BQ0210FS_PD_3X2_7LM_PU_3P3  Cell operated at 3
|BQ0210FS_PD_3X2_7LM_PU_3P3; PULLUP_ON
BQ0210FS_PD_3X2_7LM_PD_3P3  Cell operated at 3
|BQ0210FS_PD_3X2_7LM_PD_3P3; PULLDOWN_ON
[Model Selector]   BQ0210FS_PD_3X2_7LM_N4
BQ0210FS_PD_3X2_7LM_PZ_3P3  Cell operated at 3
|BQ0210FS_PD_3X2_7LM_PZ_3P3; PUPD_OFF
BQ0210FS_PD_3X2_7LM_PU_3P3  Cell operated at 3
|BQ0210FS_PD_3X2_7LM_PU_3P3; PULLUP_ON
BQ0210FS_PD_3X2_7LM_PD_3P3  Cell operated at 3
|BQ0210FS_PD_3X2_7LM_PD_3P3; PULLDOWN_ON
[Model Selector]   BQ0210FS_PD_3X2_7LM_P4
BQ0210FS_PD_3X2_7LM_PZ_3P3  Cell operated at 3
|BQ0210FS_PD_3X2_7LM_PZ_3P3; PUPD_OFF
BQ0210FS_PD_3X2_7LM_PU_3P3  Cell operated at 3
|BQ0210FS_PD_3X2_7LM_PU_3P3; PULLUP_ON
BQ0210FS_PD_3X2_7LM_PD_3P3  Cell operated at 3
|BQ0210FS_PD_3X2_7LM_PD_3P3; PULLDOWN_ON
[Model Selector]   BQ0210FS_PD_3X2_7LM_T10
BQ0210FS_PD_3X2_7LM_PZ_3P3  Cell operated at 3
|BQ0210FS_PD_3X2_7LM_PZ_3P3; PUPD_OFF
BQ0210FS_PD_3X2_7LM_PU_3P3  Cell operated at 3
|BQ0210FS_PD_3X2_7LM_PU_3P3; PULLUP_ON
BQ0210FS_PD_3X2_7LM_PD_3P3  Cell operated at 3
|BQ0210FS_PD_3X2_7LM_PD_3P3; PULLDOWN_ON
[Model Selector]   BQ0210FS_PD_3X2_7LM_T5
BQ0210FS_PD_3X2_7LM_PZ_3P3  Cell operated at 3
|BQ0210FS_PD_3X2_7LM_PZ_3P3; PUPD_OFF
BQ0210FS_PD_3X2_7LM_PU_3P3  Cell operated at 3
|BQ0210FS_PD_3X2_7LM_PU_3P3; PULLUP_ON
BQ0210FS_PD_3X2_7LM_PD_3P3  Cell operated at 3
|BQ0210FS_PD_3X2_7LM_PD_3P3; PULLDOWN_ON
[Model Selector]   BQ0210FS_PD_3X2_7LM_T6
BQ0210FS_PD_3X2_7LM_PZ_3P3  Cell operated at 3
|BQ0210FS_PD_3X2_7LM_PZ_3P3; PUPD_OFF
BQ0210FS_PD_3X2_7LM_PU_3P3  Cell operated at 3
|BQ0210FS_PD_3X2_7LM_PU_3P3; PULLUP_ON
BQ0210FS_PD_3X2_7LM_PD_3P3  Cell operated at 3
|BQ0210FS_PD_3X2_7LM_PD_3P3; PULLDOWN_ON
[Model Selector]   BQ0210FS_PD_3X2_7LM_T7
BQ0210FS_PD_3X2_7LM_PZ_3P3  Cell operated at 3
|BQ0210FS_PD_3X2_7LM_PZ_3P3; PUPD_OFF
BQ0210FS_PD_3X2_7LM_PU_3P3  Cell operated at 3
|BQ0210FS_PD_3X2_7LM_PU_3P3; PULLUP_ON
BQ0210FS_PD_3X2_7LM_PD_3P3  Cell operated at 3
|BQ0210FS_PD_3X2_7LM_PD_3P3; PULLDOWN_ON
[Model Selector]   BQ0210FS_PD_3X2_7LM_T8
BQ0210FS_PD_3X2_7LM_PZ_3P3  Cell operated at 3
|BQ0210FS_PD_3X2_7LM_PZ_3P3; PUPD_OFF
BQ0210FS_PD_3X2_7LM_PU_3P3  Cell operated at 3
|BQ0210FS_PD_3X2_7LM_PU_3P3; PULLUP_ON
BQ0210FS_PD_3X2_7LM_PD_3P3  Cell operated at 3
|BQ0210FS_PD_3X2_7LM_PD_3P3; PULLDOWN_ON
[Model Selector]   BQ0210FS_PD_3X2_7LM_W10
BQ0210FS_PD_3X2_7LM_PZ_3P3  Cell operated at 3
|BQ0210FS_PD_3X2_7LM_PZ_3P3; PUPD_OFF
BQ0210FS_PD_3X2_7LM_PU_3P3  Cell operated at 3
|BQ0210FS_PD_3X2_7LM_PU_3P3; PULLUP_ON
BQ0210FS_PD_3X2_7LM_PD_3P3  Cell operated at 3
|BQ0210FS_PD_3X2_7LM_PD_3P3; PULLDOWN_ON
[Model Selector]   BQ0210FS_PD_3X2_V2_7LM_D3
BQ0210FS_PD_3X2_V2_7LM_PZ_3P3  Cell operated at 3
|BQ0210FS_PD_3X2_V2_7LM_PZ_3P3; PUPD_OFF
BQ0210FS_PD_3X2_V2_7LM_PU_3P3  Cell operated at 3
|BQ0210FS_PD_3X2_V2_7LM_PU_3P3; PULLUP_ON
BQ0210FS_PD_3X2_V2_7LM_PD_3P3  Cell operated at 3
|BQ0210FS_PD_3X2_V2_7LM_PD_3P3; PULLDOWN_ON
[Model Selector]   BQ0210FS_PD_3X2_V2_7LM_E3
BQ0210FS_PD_3X2_V2_7LM_PZ_3P3  Cell operated at 3
|BQ0210FS_PD_3X2_V2_7LM_PZ_3P3; PUPD_OFF
BQ0210FS_PD_3X2_V2_7LM_PU_3P3  Cell operated at 3
|BQ0210FS_PD_3X2_V2_7LM_PU_3P3; PULLUP_ON
BQ0210FS_PD_3X2_V2_7LM_PD_3P3  Cell operated at 3
|BQ0210FS_PD_3X2_V2_7LM_PD_3P3; PULLDOWN_ON
[Model Selector]   BQ0210FS_PD_3X2_V2_7LM_N3
BQ0210FS_PD_3X2_V2_7LM_PZ_3P3  Cell operated at 3
|BQ0210FS_PD_3X2_V2_7LM_PZ_3P3; PUPD_OFF
BQ0210FS_PD_3X2_V2_7LM_PU_3P3  Cell operated at 3
|BQ0210FS_PD_3X2_V2_7LM_PU_3P3; PULLUP_ON
BQ0210FS_PD_3X2_V2_7LM_PD_3P3  Cell operated at 3
|BQ0210FS_PD_3X2_V2_7LM_PD_3P3; PULLDOWN_ON
[Model Selector]   BQ0210FS_PD_3X2_V2_7LM_P1
BQ0210FS_PD_3X2_V2_7LM_PZ_3P3  Cell operated at 3
|BQ0210FS_PD_3X2_V2_7LM_PZ_3P3; PUPD_OFF
BQ0210FS_PD_3X2_V2_7LM_PU_3P3  Cell operated at 3
|BQ0210FS_PD_3X2_V2_7LM_PU_3P3; PULLUP_ON
BQ0210FS_PD_3X2_V2_7LM_PD_3P3  Cell operated at 3
|BQ0210FS_PD_3X2_V2_7LM_PD_3P3; PULLDOWN_ON
[Model Selector]   BQ0210FS_PD_3X2_V2_7LM_U1
BQ0210FS_PD_3X2_V2_7LM_PZ_3P3  Cell operated at 3
|BQ0210FS_PD_3X2_V2_7LM_PZ_3P3; PUPD_OFF
BQ0210FS_PD_3X2_V2_7LM_PU_3P3  Cell operated at 3
|BQ0210FS_PD_3X2_V2_7LM_PU_3P3; PULLUP_ON
BQ0210FS_PD_3X2_V2_7LM_PD_3P3  Cell operated at 3
|BQ0210FS_PD_3X2_V2_7LM_PD_3P3; PULLDOWN_ON
[Model Selector]   BQ0210FS_PU_3X2_7LM_A10
BQ0210FS_PU_3X2_7LM_PZ_3P3  Cell operated at 3
|BQ0210FS_PU_3X2_7LM_PZ_3P3; PUPD_OFF
BQ0210FS_PU_3X2_7LM_PU_3P3  Cell operated at 3
|BQ0210FS_PU_3X2_7LM_PU_3P3; PULLUP_ON
BQ0210FS_PU_3X2_7LM_PD_3P3  Cell operated at 3
|BQ0210FS_PU_3X2_7LM_PD_3P3; PULLDOWN_ON
[Model Selector]   BQ0210FS_PU_3X2_7LM_A7
BQ0210FS_PU_3X2_7LM_PZ_3P3  Cell operated at 3
|BQ0210FS_PU_3X2_7LM_PZ_3P3; PUPD_OFF
BQ0210FS_PU_3X2_7LM_PU_3P3  Cell operated at 3
|BQ0210FS_PU_3X2_7LM_PU_3P3; PULLUP_ON
BQ0210FS_PU_3X2_7LM_PD_3P3  Cell operated at 3
|BQ0210FS_PU_3X2_7LM_PD_3P3; PULLDOWN_ON
[Model Selector]   BQ0210FS_PU_3X2_7LM_B10
BQ0210FS_PU_3X2_7LM_PZ_3P3  Cell operated at 3
|BQ0210FS_PU_3X2_7LM_PZ_3P3; PUPD_OFF
BQ0210FS_PU_3X2_7LM_PU_3P3  Cell operated at 3
|BQ0210FS_PU_3X2_7LM_PU_3P3; PULLUP_ON
BQ0210FS_PU_3X2_7LM_PD_3P3  Cell operated at 3
|BQ0210FS_PU_3X2_7LM_PD_3P3; PULLDOWN_ON
[Model Selector]   BQ0210FS_PU_3X2_7LM_B7
BQ0210FS_PU_3X2_7LM_PZ_3P3  Cell operated at 3
|BQ0210FS_PU_3X2_7LM_PZ_3P3; PUPD_OFF
BQ0210FS_PU_3X2_7LM_PU_3P3  Cell operated at 3
|BQ0210FS_PU_3X2_7LM_PU_3P3; PULLUP_ON
BQ0210FS_PU_3X2_7LM_PD_3P3  Cell operated at 3
|BQ0210FS_PU_3X2_7LM_PD_3P3; PULLDOWN_ON
[Model Selector]   BQ0210FS_PU_3X2_7LM_F16
BQ0210FS_PU_3X2_7LM_PZ_3P3  Cell operated at 3
|BQ0210FS_PU_3X2_7LM_PZ_3P3; PUPD_OFF
BQ0210FS_PU_3X2_7LM_PU_3P3  Cell operated at 3
|BQ0210FS_PU_3X2_7LM_PU_3P3; PULLUP_ON
BQ0210FS_PU_3X2_7LM_PD_3P3  Cell operated at 3
|BQ0210FS_PU_3X2_7LM_PD_3P3; PULLDOWN_ON
[Model Selector]   BQ0210FS_PU_3X2_7LM_F17
BQ0210FS_PU_3X2_7LM_PZ_3P3  Cell operated at 3
|BQ0210FS_PU_3X2_7LM_PZ_3P3; PUPD_OFF
BQ0210FS_PU_3X2_7LM_PU_3P3  Cell operated at 3
|BQ0210FS_PU_3X2_7LM_PU_3P3; PULLUP_ON
BQ0210FS_PU_3X2_7LM_PD_3P3  Cell operated at 3
|BQ0210FS_PU_3X2_7LM_PD_3P3; PULLDOWN_ON
[Model Selector]   BQ0210FS_PU_3X2_7LM_H1
BQ0210FS_PU_3X2_7LM_PZ_3P3  Cell operated at 3
|BQ0210FS_PU_3X2_7LM_PZ_3P3; PUPD_OFF
BQ0210FS_PU_3X2_7LM_PU_3P3  Cell operated at 3
|BQ0210FS_PU_3X2_7LM_PU_3P3; PULLUP_ON
BQ0210FS_PU_3X2_7LM_PD_3P3  Cell operated at 3
|BQ0210FS_PU_3X2_7LM_PD_3P3; PULLDOWN_ON
[Model Selector]   BQ0210FS_PU_3X2_7LM_H2
BQ0210FS_PU_3X2_7LM_PZ_3P3  Cell operated at 3
|BQ0210FS_PU_3X2_7LM_PZ_3P3; PUPD_OFF
BQ0210FS_PU_3X2_7LM_PU_3P3  Cell operated at 3
|BQ0210FS_PU_3X2_7LM_PU_3P3; PULLUP_ON
BQ0210FS_PU_3X2_7LM_PD_3P3  Cell operated at 3
|BQ0210FS_PU_3X2_7LM_PD_3P3; PULLDOWN_ON
[Model Selector]   BQ0210FS_PU_3X2_7LM_J16
BQ0210FS_PU_3X2_7LM_PZ_3P3  Cell operated at 3
|BQ0210FS_PU_3X2_7LM_PZ_3P3; PUPD_OFF
BQ0210FS_PU_3X2_7LM_PU_3P3  Cell operated at 3
|BQ0210FS_PU_3X2_7LM_PU_3P3; PULLUP_ON
BQ0210FS_PU_3X2_7LM_PD_3P3  Cell operated at 3
|BQ0210FS_PU_3X2_7LM_PD_3P3; PULLDOWN_ON
[Model Selector]   BQ0210FS_PU_3X2_7LM_L18
BQ0210FS_PU_3X2_7LM_PZ_3P3  Cell operated at 3
|BQ0210FS_PU_3X2_7LM_PZ_3P3; PUPD_OFF
BQ0210FS_PU_3X2_7LM_PU_3P3  Cell operated at 3
|BQ0210FS_PU_3X2_7LM_PU_3P3; PULLUP_ON
BQ0210FS_PU_3X2_7LM_PD_3P3  Cell operated at 3
|BQ0210FS_PU_3X2_7LM_PD_3P3; PULLDOWN_ON
[Model Selector]   BQ0210FS_PU_3X2_7LM_L19
BQ0210FS_PU_3X2_7LM_PZ_3P3  Cell operated at 3
|BQ0210FS_PU_3X2_7LM_PZ_3P3; PUPD_OFF
BQ0210FS_PU_3X2_7LM_PU_3P3  Cell operated at 3
|BQ0210FS_PU_3X2_7LM_PU_3P3; PULLUP_ON
BQ0210FS_PU_3X2_7LM_PD_3P3  Cell operated at 3
|BQ0210FS_PU_3X2_7LM_PD_3P3; PULLDOWN_ON
[Model Selector]   BQ0210FS_PU_3X2_7LM_M18
BQ0210FS_PU_3X2_7LM_PZ_3P3  Cell operated at 3
|BQ0210FS_PU_3X2_7LM_PZ_3P3; PUPD_OFF
BQ0210FS_PU_3X2_7LM_PU_3P3  Cell operated at 3
|BQ0210FS_PU_3X2_7LM_PU_3P3; PULLUP_ON
BQ0210FS_PU_3X2_7LM_PD_3P3  Cell operated at 3
|BQ0210FS_PU_3X2_7LM_PD_3P3; PULLDOWN_ON
[Model Selector]   BQ0210FS_PU_3X2_7LM_M19
BQ0210FS_PU_3X2_7LM_PZ_3P3  Cell operated at 3
|BQ0210FS_PU_3X2_7LM_PZ_3P3; PUPD_OFF
BQ0210FS_PU_3X2_7LM_PU_3P3  Cell operated at 3
|BQ0210FS_PU_3X2_7LM_PU_3P3; PULLUP_ON
BQ0210FS_PU_3X2_7LM_PD_3P3  Cell operated at 3
|BQ0210FS_PU_3X2_7LM_PD_3P3; PULLDOWN_ON
[Model Selector]   BQ0210FS_PU_3X2_7LM_P3
BQ0210FS_PU_3X2_7LM_PZ_3P3  Cell operated at 3
|BQ0210FS_PU_3X2_7LM_PZ_3P3; PUPD_OFF
BQ0210FS_PU_3X2_7LM_PU_3P3  Cell operated at 3
|BQ0210FS_PU_3X2_7LM_PU_3P3; PULLUP_ON
BQ0210FS_PU_3X2_7LM_PD_3P3  Cell operated at 3
|BQ0210FS_PU_3X2_7LM_PD_3P3; PULLDOWN_ON
[Model Selector]   BQ0210FS_PU_3X2_7LM_R9
BQ0210FS_PU_3X2_7LM_PZ_3P3  Cell operated at 3
|BQ0210FS_PU_3X2_7LM_PZ_3P3; PUPD_OFF
BQ0210FS_PU_3X2_7LM_PU_3P3  Cell operated at 3
|BQ0210FS_PU_3X2_7LM_PU_3P3; PULLUP_ON
BQ0210FS_PU_3X2_7LM_PD_3P3  Cell operated at 3
|BQ0210FS_PU_3X2_7LM_PD_3P3; PULLDOWN_ON
[Model Selector]   BQ0210FS_PU_3X2_V2_7LM_B2
BQ0210FS_PU_3X2_V2_7LM_PZ_3P3  Cell operated at 3
|BQ0210FS_PU_3X2_V2_7LM_PZ_3P3; PUPD_OFF
BQ0210FS_PU_3X2_V2_7LM_PU_3P3  Cell operated at 3
|BQ0210FS_PU_3X2_V2_7LM_PU_3P3; PULLUP_ON
BQ0210FS_PU_3X2_V2_7LM_PD_3P3  Cell operated at 3
|BQ0210FS_PU_3X2_V2_7LM_PD_3P3; PULLDOWN_ON
[Model Selector]   BQ0210FS_PU_3X2_V2_7LM_B6
BQ0210FS_PU_3X2_V2_7LM_PZ_3P3  Cell operated at 3
|BQ0210FS_PU_3X2_V2_7LM_PZ_3P3; PUPD_OFF
BQ0210FS_PU_3X2_V2_7LM_PU_3P3  Cell operated at 3
|BQ0210FS_PU_3X2_V2_7LM_PU_3P3; PULLUP_ON
BQ0210FS_PU_3X2_V2_7LM_PD_3P3  Cell operated at 3
|BQ0210FS_PU_3X2_V2_7LM_PD_3P3; PULLDOWN_ON
[Model Selector]   BQ0210FS_PU_3X2_V2_7LM_C3
BQ0210FS_PU_3X2_V2_7LM_PZ_3P3  Cell operated at 3
|BQ0210FS_PU_3X2_V2_7LM_PZ_3P3; PUPD_OFF
BQ0210FS_PU_3X2_V2_7LM_PU_3P3  Cell operated at 3
|BQ0210FS_PU_3X2_V2_7LM_PU_3P3; PULLUP_ON
BQ0210FS_PU_3X2_V2_7LM_PD_3P3  Cell operated at 3
|BQ0210FS_PU_3X2_V2_7LM_PD_3P3; PULLDOWN_ON
[Model Selector]   BQ0210FS_PU_3X2_V2_7LM_J3
BQ0210FS_PU_3X2_V2_7LM_PZ_3P3  Cell operated at 3
|BQ0210FS_PU_3X2_V2_7LM_PZ_3P3; PUPD_OFF
BQ0210FS_PU_3X2_V2_7LM_PU_3P3  Cell operated at 3
|BQ0210FS_PU_3X2_V2_7LM_PU_3P3; PULLUP_ON
BQ0210FS_PU_3X2_V2_7LM_PD_3P3  Cell operated at 3
|BQ0210FS_PU_3X2_V2_7LM_PD_3P3; PULLDOWN_ON
[Model Selector]   BQ0210FS_PU_3X2_V2_7LM_T12
BQ0210FS_PU_3X2_V2_7LM_PZ_3P3  Cell operated at 3
|BQ0210FS_PU_3X2_V2_7LM_PZ_3P3; PUPD_OFF
BQ0210FS_PU_3X2_V2_7LM_PU_3P3  Cell operated at 3
|BQ0210FS_PU_3X2_V2_7LM_PU_3P3; PULLUP_ON
BQ0210FS_PU_3X2_V2_7LM_PD_3P3  Cell operated at 3
|BQ0210FS_PU_3X2_V2_7LM_PD_3P3; PULLDOWN_ON
[Model Selector]   BQ0210FS_PU_3X2_V2_7LM_U10
BQ0210FS_PU_3X2_V2_7LM_PZ_3P3  Cell operated at 3
|BQ0210FS_PU_3X2_V2_7LM_PZ_3P3; PUPD_OFF
BQ0210FS_PU_3X2_V2_7LM_PU_3P3  Cell operated at 3
|BQ0210FS_PU_3X2_V2_7LM_PU_3P3; PULLUP_ON
BQ0210FS_PU_3X2_V2_7LM_PD_3P3  Cell operated at 3
|BQ0210FS_PU_3X2_V2_7LM_PD_3P3; PULLDOWN_ON
[Model Selector]   BQ0210FS_PU_3X2_V2_7LM_U9
BQ0210FS_PU_3X2_V2_7LM_PZ_3P3  Cell operated at 3
|BQ0210FS_PU_3X2_V2_7LM_PZ_3P3; PUPD_OFF
BQ0210FS_PU_3X2_V2_7LM_PU_3P3  Cell operated at 3
|BQ0210FS_PU_3X2_V2_7LM_PU_3P3; PULLUP_ON
BQ0210FS_PU_3X2_V2_7LM_PD_3P3  Cell operated at 3
|BQ0210FS_PU_3X2_V2_7LM_PD_3P3; PULLDOWN_ON
[Model Selector]   BQ0210FS_PU_3X2_V2_7LM_W6
BQ0210FS_PU_3X2_V2_7LM_PZ_3P3  Cell operated at 3
|BQ0210FS_PU_3X2_V2_7LM_PZ_3P3; PUPD_OFF
BQ0210FS_PU_3X2_V2_7LM_PU_3P3  Cell operated at 3
|BQ0210FS_PU_3X2_V2_7LM_PU_3P3; PULLUP_ON
BQ0210FS_PU_3X2_V2_7LM_PD_3P3  Cell operated at 3
|BQ0210FS_PU_3X2_V2_7LM_PD_3P3; PULLDOWN_ON
[Model Selector]   BQ0210FS_PU_3X2_V2_7LM_W9
BQ0210FS_PU_3X2_V2_7LM_PZ_3P3  Cell operated at 3
|BQ0210FS_PU_3X2_V2_7LM_PZ_3P3; PUPD_OFF
BQ0210FS_PU_3X2_V2_7LM_PU_3P3  Cell operated at 3
|BQ0210FS_PU_3X2_V2_7LM_PU_3P3; PULLUP_ON
BQ0210FS_PU_3X2_V2_7LM_PD_3P3  Cell operated at 3
|BQ0210FS_PU_3X2_V2_7LM_PD_3P3; PULLDOWN_ON
[Model Selector]   BQ0212FS_3X2_7LM_A16
BQ0212FS_3X2_7LM_PZ_3P3  Cell operated at 3
|BQ0212FS_3X2_7LM_PZ_3P3; PUPD_OFF
BQ0212FS_3X2_7LM_PU_3P3  Cell operated at 3
|BQ0212FS_3X2_7LM_PU_3P3; PULLUP_ON
BQ0212FS_3X2_7LM_PD_3P3  Cell operated at 3
|BQ0212FS_3X2_7LM_PD_3P3; PULLDOWN_ON
[Model Selector]   BQ0212FS_3X2_7LM_D10
BQ0212FS_3X2_7LM_PZ_3P3  Cell operated at 3
|BQ0212FS_3X2_7LM_PZ_3P3; PUPD_OFF
BQ0212FS_3X2_7LM_PU_3P3  Cell operated at 3
|BQ0212FS_3X2_7LM_PU_3P3; PULLUP_ON
BQ0212FS_3X2_7LM_PD_3P3  Cell operated at 3
|BQ0212FS_3X2_7LM_PD_3P3; PULLDOWN_ON
[Model Selector]   BQ0212FS_3X2_7LM_D17
BQ0212FS_3X2_7LM_PZ_3P3  Cell operated at 3
|BQ0212FS_3X2_7LM_PZ_3P3; PUPD_OFF
BQ0212FS_3X2_7LM_PU_3P3  Cell operated at 3
|BQ0212FS_3X2_7LM_PU_3P3; PULLUP_ON
BQ0212FS_3X2_7LM_PD_3P3  Cell operated at 3
|BQ0212FS_3X2_7LM_PD_3P3; PULLDOWN_ON
[Model Selector]   BQ0212FS_3X2_7LM_D9
BQ0212FS_3X2_7LM_PZ_3P3  Cell operated at 3
|BQ0212FS_3X2_7LM_PZ_3P3; PUPD_OFF
BQ0212FS_3X2_7LM_PU_3P3  Cell operated at 3
|BQ0212FS_3X2_7LM_PU_3P3; PULLUP_ON
BQ0212FS_3X2_7LM_PD_3P3  Cell operated at 3
|BQ0212FS_3X2_7LM_PD_3P3; PULLDOWN_ON
[Model Selector]   BQ0212FS_3X2_7LM_E4
BQ0212FS_3X2_7LM_PZ_3P3  Cell operated at 3
|BQ0212FS_3X2_7LM_PZ_3P3; PUPD_OFF
BQ0212FS_3X2_7LM_PU_3P3  Cell operated at 3
|BQ0212FS_3X2_7LM_PU_3P3; PULLUP_ON
BQ0212FS_3X2_7LM_PD_3P3  Cell operated at 3
|BQ0212FS_3X2_7LM_PD_3P3; PULLDOWN_ON
[Model Selector]   BQ0212FS_3X2_7LM_G4
BQ0212FS_3X2_7LM_PZ_3P3  Cell operated at 3
|BQ0212FS_3X2_7LM_PZ_3P3; PUPD_OFF
BQ0212FS_3X2_7LM_PU_3P3  Cell operated at 3
|BQ0212FS_3X2_7LM_PU_3P3; PULLUP_ON
BQ0212FS_3X2_7LM_PD_3P3  Cell operated at 3
|BQ0212FS_3X2_7LM_PD_3P3; PULLDOWN_ON
[Model Selector]   BQ0212FS_3X2_7LM_L3
BQ0212FS_3X2_7LM_PZ_3P3  Cell operated at 3
|BQ0212FS_3X2_7LM_PZ_3P3; PUPD_OFF
BQ0212FS_3X2_7LM_PU_3P3  Cell operated at 3
|BQ0212FS_3X2_7LM_PU_3P3; PULLUP_ON
BQ0212FS_3X2_7LM_PD_3P3  Cell operated at 3
|BQ0212FS_3X2_7LM_PD_3P3; PULLDOWN_ON
[Model Selector]   BQ0212FS_3X2_7LM_R1
BQ0212FS_3X2_7LM_PZ_3P3  Cell operated at 3
|BQ0212FS_3X2_7LM_PZ_3P3; PUPD_OFF
BQ0212FS_3X2_7LM_PU_3P3  Cell operated at 3
|BQ0212FS_3X2_7LM_PU_3P3; PULLUP_ON
BQ0212FS_3X2_7LM_PD_3P3  Cell operated at 3
|BQ0212FS_3X2_7LM_PD_3P3; PULLDOWN_ON
[Model Selector]   BQ0212FS_3X2_7LM_T2
BQ0212FS_3X2_7LM_PZ_3P3  Cell operated at 3
|BQ0212FS_3X2_7LM_PZ_3P3; PUPD_OFF
BQ0212FS_3X2_7LM_PU_3P3  Cell operated at 3
|BQ0212FS_3X2_7LM_PU_3P3; PULLUP_ON
BQ0212FS_3X2_7LM_PD_3P3  Cell operated at 3
|BQ0212FS_3X2_7LM_PD_3P3; PULLDOWN_ON
[Model Selector]   BQ0212FS_3X2_7LM_T9
BQ0212FS_3X2_7LM_PZ_3P3  Cell operated at 3
|BQ0212FS_3X2_7LM_PZ_3P3; PUPD_OFF
BQ0212FS_3X2_7LM_PU_3P3  Cell operated at 3
|BQ0212FS_3X2_7LM_PU_3P3; PULLUP_ON
BQ0212FS_3X2_7LM_PD_3P3  Cell operated at 3
|BQ0212FS_3X2_7LM_PD_3P3; PULLDOWN_ON
[Model Selector]   BQ0212FS_3X2_7LM_U8
BQ0212FS_3X2_7LM_PZ_3P3  Cell operated at 3
|BQ0212FS_3X2_7LM_PZ_3P3; PUPD_OFF
BQ0212FS_3X2_7LM_PU_3P3  Cell operated at 3
|BQ0212FS_3X2_7LM_PU_3P3; PULLUP_ON
BQ0212FS_3X2_7LM_PD_3P3  Cell operated at 3
|BQ0212FS_3X2_7LM_PD_3P3; PULLDOWN_ON
[Model Selector]   BQ0212FS_PD_3X2_7LM_B14
BQ0212FS_PD_3X2_7LM_PZ_3P3  Cell operated at 3
|BQ0212FS_PD_3X2_7LM_PZ_3P3; PUPD_OFF
BQ0212FS_PD_3X2_7LM_PU_3P3  Cell operated at 3
|BQ0212FS_PD_3X2_7LM_PU_3P3; PULLUP_ON
BQ0212FS_PD_3X2_7LM_PD_3P3  Cell operated at 3
|BQ0212FS_PD_3X2_7LM_PD_3P3; PULLDOWN_ON
[Model Selector]   BQ0212FS_PD_3X2_7LM_C10
BQ0212FS_PD_3X2_7LM_PZ_3P3  Cell operated at 3
|BQ0212FS_PD_3X2_7LM_PZ_3P3; PUPD_OFF
BQ0212FS_PD_3X2_7LM_PU_3P3  Cell operated at 3
|BQ0212FS_PD_3X2_7LM_PU_3P3; PULLUP_ON
BQ0212FS_PD_3X2_7LM_PD_3P3  Cell operated at 3
|BQ0212FS_PD_3X2_7LM_PD_3P3; PULLDOWN_ON
[Model Selector]   BQ0212FS_PD_3X2_7LM_C11
BQ0212FS_PD_3X2_7LM_PZ_3P3  Cell operated at 3
|BQ0212FS_PD_3X2_7LM_PZ_3P3; PUPD_OFF
BQ0212FS_PD_3X2_7LM_PU_3P3  Cell operated at 3
|BQ0212FS_PD_3X2_7LM_PU_3P3; PULLUP_ON
BQ0212FS_PD_3X2_7LM_PD_3P3  Cell operated at 3
|BQ0212FS_PD_3X2_7LM_PD_3P3; PULLDOWN_ON
[Model Selector]   BQ0212FS_PD_3X2_7LM_C12
BQ0212FS_PD_3X2_7LM_PZ_3P3  Cell operated at 3
|BQ0212FS_PD_3X2_7LM_PZ_3P3; PUPD_OFF
BQ0212FS_PD_3X2_7LM_PU_3P3  Cell operated at 3
|BQ0212FS_PD_3X2_7LM_PU_3P3; PULLUP_ON
BQ0212FS_PD_3X2_7LM_PD_3P3  Cell operated at 3
|BQ0212FS_PD_3X2_7LM_PD_3P3; PULLDOWN_ON
[Model Selector]   BQ0212FS_PD_3X2_7LM_C13
BQ0212FS_PD_3X2_7LM_PZ_3P3  Cell operated at 3
|BQ0212FS_PD_3X2_7LM_PZ_3P3; PUPD_OFF
BQ0212FS_PD_3X2_7LM_PU_3P3  Cell operated at 3
|BQ0212FS_PD_3X2_7LM_PU_3P3; PULLUP_ON
BQ0212FS_PD_3X2_7LM_PD_3P3  Cell operated at 3
|BQ0212FS_PD_3X2_7LM_PD_3P3; PULLDOWN_ON
[Model Selector]   BQ0212FS_PD_3X2_7LM_C14
BQ0212FS_PD_3X2_7LM_PZ_3P3  Cell operated at 3
|BQ0212FS_PD_3X2_7LM_PZ_3P3; PUPD_OFF
BQ0212FS_PD_3X2_7LM_PU_3P3  Cell operated at 3
|BQ0212FS_PD_3X2_7LM_PU_3P3; PULLUP_ON
BQ0212FS_PD_3X2_7LM_PD_3P3  Cell operated at 3
|BQ0212FS_PD_3X2_7LM_PD_3P3; PULLDOWN_ON
[Model Selector]   BQ0212FS_PD_3X2_7LM_C17
BQ0212FS_PD_3X2_7LM_PZ_3P3  Cell operated at 3
|BQ0212FS_PD_3X2_7LM_PZ_3P3; PUPD_OFF
BQ0212FS_PD_3X2_7LM_PU_3P3  Cell operated at 3
|BQ0212FS_PD_3X2_7LM_PU_3P3; PULLUP_ON
BQ0212FS_PD_3X2_7LM_PD_3P3  Cell operated at 3
|BQ0212FS_PD_3X2_7LM_PD_3P3; PULLDOWN_ON
[Model Selector]   BQ0212FS_PD_3X2_7LM_C7
BQ0212FS_PD_3X2_7LM_PZ_3P3  Cell operated at 3
|BQ0212FS_PD_3X2_7LM_PZ_3P3; PUPD_OFF
BQ0212FS_PD_3X2_7LM_PU_3P3  Cell operated at 3
|BQ0212FS_PD_3X2_7LM_PU_3P3; PULLUP_ON
BQ0212FS_PD_3X2_7LM_PD_3P3  Cell operated at 3
|BQ0212FS_PD_3X2_7LM_PD_3P3; PULLDOWN_ON
[Model Selector]   BQ0212FS_PD_3X2_7LM_C8
BQ0212FS_PD_3X2_7LM_PZ_3P3  Cell operated at 3
|BQ0212FS_PD_3X2_7LM_PZ_3P3; PUPD_OFF
BQ0212FS_PD_3X2_7LM_PU_3P3  Cell operated at 3
|BQ0212FS_PD_3X2_7LM_PU_3P3; PULLUP_ON
BQ0212FS_PD_3X2_7LM_PD_3P3  Cell operated at 3
|BQ0212FS_PD_3X2_7LM_PD_3P3; PULLDOWN_ON
[Model Selector]   BQ0212FS_PD_3X2_7LM_C9
BQ0212FS_PD_3X2_7LM_PZ_3P3  Cell operated at 3
|BQ0212FS_PD_3X2_7LM_PZ_3P3; PUPD_OFF
BQ0212FS_PD_3X2_7LM_PU_3P3  Cell operated at 3
|BQ0212FS_PD_3X2_7LM_PU_3P3; PULLUP_ON
BQ0212FS_PD_3X2_7LM_PD_3P3  Cell operated at 3
|BQ0212FS_PD_3X2_7LM_PD_3P3; PULLDOWN_ON
[Model Selector]   BQ0212FS_PD_3X2_7LM_D14
BQ0212FS_PD_3X2_7LM_PZ_3P3  Cell operated at 3
|BQ0212FS_PD_3X2_7LM_PZ_3P3; PUPD_OFF
BQ0212FS_PD_3X2_7LM_PU_3P3  Cell operated at 3
|BQ0212FS_PD_3X2_7LM_PU_3P3; PULLUP_ON
BQ0212FS_PD_3X2_7LM_PD_3P3  Cell operated at 3
|BQ0212FS_PD_3X2_7LM_PD_3P3; PULLDOWN_ON
[Model Selector]   BQ0212FS_PD_3X2_7LM_D15
BQ0212FS_PD_3X2_7LM_PZ_3P3  Cell operated at 3
|BQ0212FS_PD_3X2_7LM_PZ_3P3; PUPD_OFF
BQ0212FS_PD_3X2_7LM_PU_3P3  Cell operated at 3
|BQ0212FS_PD_3X2_7LM_PU_3P3; PULLUP_ON
BQ0212FS_PD_3X2_7LM_PD_3P3  Cell operated at 3
|BQ0212FS_PD_3X2_7LM_PD_3P3; PULLDOWN_ON
[Model Selector]   BQ0212FS_PD_3X2_7LM_E10
BQ0212FS_PD_3X2_7LM_PZ_3P3  Cell operated at 3
|BQ0212FS_PD_3X2_7LM_PZ_3P3; PUPD_OFF
BQ0212FS_PD_3X2_7LM_PU_3P3  Cell operated at 3
|BQ0212FS_PD_3X2_7LM_PU_3P3; PULLUP_ON
BQ0212FS_PD_3X2_7LM_PD_3P3  Cell operated at 3
|BQ0212FS_PD_3X2_7LM_PD_3P3; PULLDOWN_ON
[Model Selector]   BQ0212FS_PD_3X2_7LM_E11
BQ0212FS_PD_3X2_7LM_PZ_3P3  Cell operated at 3
|BQ0212FS_PD_3X2_7LM_PZ_3P3; PUPD_OFF
BQ0212FS_PD_3X2_7LM_PU_3P3  Cell operated at 3
|BQ0212FS_PD_3X2_7LM_PU_3P3; PULLUP_ON
BQ0212FS_PD_3X2_7LM_PD_3P3  Cell operated at 3
|BQ0212FS_PD_3X2_7LM_PD_3P3; PULLDOWN_ON
[Model Selector]   BQ0212FS_PD_3X2_7LM_E12
BQ0212FS_PD_3X2_7LM_PZ_3P3  Cell operated at 3
|BQ0212FS_PD_3X2_7LM_PZ_3P3; PUPD_OFF
BQ0212FS_PD_3X2_7LM_PU_3P3  Cell operated at 3
|BQ0212FS_PD_3X2_7LM_PU_3P3; PULLUP_ON
BQ0212FS_PD_3X2_7LM_PD_3P3  Cell operated at 3
|BQ0212FS_PD_3X2_7LM_PD_3P3; PULLDOWN_ON
[Model Selector]   BQ0212FS_PD_3X2_7LM_E13
BQ0212FS_PD_3X2_7LM_PZ_3P3  Cell operated at 3
|BQ0212FS_PD_3X2_7LM_PZ_3P3; PUPD_OFF
BQ0212FS_PD_3X2_7LM_PU_3P3  Cell operated at 3
|BQ0212FS_PD_3X2_7LM_PU_3P3; PULLUP_ON
BQ0212FS_PD_3X2_7LM_PD_3P3  Cell operated at 3
|BQ0212FS_PD_3X2_7LM_PD_3P3; PULLDOWN_ON
[Model Selector]   BQ0212FS_PD_3X2_7LM_E14
BQ0212FS_PD_3X2_7LM_PZ_3P3  Cell operated at 3
|BQ0212FS_PD_3X2_7LM_PZ_3P3; PUPD_OFF
BQ0212FS_PD_3X2_7LM_PU_3P3  Cell operated at 3
|BQ0212FS_PD_3X2_7LM_PU_3P3; PULLUP_ON
BQ0212FS_PD_3X2_7LM_PD_3P3  Cell operated at 3
|BQ0212FS_PD_3X2_7LM_PD_3P3; PULLDOWN_ON
[Model Selector]   BQ0212FS_PD_3X2_7LM_E15
BQ0212FS_PD_3X2_7LM_PZ_3P3  Cell operated at 3
|BQ0212FS_PD_3X2_7LM_PZ_3P3; PUPD_OFF
BQ0212FS_PD_3X2_7LM_PU_3P3  Cell operated at 3
|BQ0212FS_PD_3X2_7LM_PU_3P3; PULLUP_ON
BQ0212FS_PD_3X2_7LM_PD_3P3  Cell operated at 3
|BQ0212FS_PD_3X2_7LM_PD_3P3; PULLDOWN_ON
[Model Selector]   BQ0212FS_PD_3X2_7LM_E5
BQ0212FS_PD_3X2_7LM_PZ_3P3  Cell operated at 3
|BQ0212FS_PD_3X2_7LM_PZ_3P3; PUPD_OFF
BQ0212FS_PD_3X2_7LM_PU_3P3  Cell operated at 3
|BQ0212FS_PD_3X2_7LM_PU_3P3; PULLUP_ON
BQ0212FS_PD_3X2_7LM_PD_3P3  Cell operated at 3
|BQ0212FS_PD_3X2_7LM_PD_3P3; PULLDOWN_ON
[Model Selector]   BQ0212FS_PD_3X2_7LM_E6
BQ0212FS_PD_3X2_7LM_PZ_3P3  Cell operated at 3
|BQ0212FS_PD_3X2_7LM_PZ_3P3; PUPD_OFF
BQ0212FS_PD_3X2_7LM_PU_3P3  Cell operated at 3
|BQ0212FS_PD_3X2_7LM_PU_3P3; PULLUP_ON
BQ0212FS_PD_3X2_7LM_PD_3P3  Cell operated at 3
|BQ0212FS_PD_3X2_7LM_PD_3P3; PULLDOWN_ON
[Model Selector]   BQ0212FS_PD_3X2_7LM_E7
BQ0212FS_PD_3X2_7LM_PZ_3P3  Cell operated at 3
|BQ0212FS_PD_3X2_7LM_PZ_3P3; PUPD_OFF
BQ0212FS_PD_3X2_7LM_PU_3P3  Cell operated at 3
|BQ0212FS_PD_3X2_7LM_PU_3P3; PULLUP_ON
BQ0212FS_PD_3X2_7LM_PD_3P3  Cell operated at 3
|BQ0212FS_PD_3X2_7LM_PD_3P3; PULLDOWN_ON
[Model Selector]   BQ0212FS_PD_3X2_7LM_E8
BQ0212FS_PD_3X2_7LM_PZ_3P3  Cell operated at 3
|BQ0212FS_PD_3X2_7LM_PZ_3P3; PUPD_OFF
BQ0212FS_PD_3X2_7LM_PU_3P3  Cell operated at 3
|BQ0212FS_PD_3X2_7LM_PU_3P3; PULLUP_ON
BQ0212FS_PD_3X2_7LM_PD_3P3  Cell operated at 3
|BQ0212FS_PD_3X2_7LM_PD_3P3; PULLDOWN_ON
[Model Selector]   BQ0212FS_PD_3X2_7LM_E9
BQ0212FS_PD_3X2_7LM_PZ_3P3  Cell operated at 3
|BQ0212FS_PD_3X2_7LM_PZ_3P3; PUPD_OFF
BQ0212FS_PD_3X2_7LM_PU_3P3  Cell operated at 3
|BQ0212FS_PD_3X2_7LM_PU_3P3; PULLUP_ON
BQ0212FS_PD_3X2_7LM_PD_3P3  Cell operated at 3
|BQ0212FS_PD_3X2_7LM_PD_3P3; PULLDOWN_ON
[Model Selector]   BQ0212FS_PD_3X2_7LM_F15
BQ0212FS_PD_3X2_7LM_PZ_3P3  Cell operated at 3
|BQ0212FS_PD_3X2_7LM_PZ_3P3; PUPD_OFF
BQ0212FS_PD_3X2_7LM_PU_3P3  Cell operated at 3
|BQ0212FS_PD_3X2_7LM_PU_3P3; PULLUP_ON
BQ0212FS_PD_3X2_7LM_PD_3P3  Cell operated at 3
|BQ0212FS_PD_3X2_7LM_PD_3P3; PULLDOWN_ON
[Model Selector]   BQ0212FS_PD_3X2_7LM_F4
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| Models and submodels in the file (58): BQ0192FS_PD_3X2_7LM_PZ_3P3 (I/O), BQ0192FS_PD_3X2_7LM_PU_3P3 (I/O), BQ0192FS_PD_3X2_7LM_PD_3P3 (I/O), BQ0192FS_PU_3X2_7LM_PZ_3P3 (I/O), BQ0192FS_PU_3X2_7LM_PU_3P3 (I/O), BQ0192FS_PU_3X2_7LM_PD_3P3 (I/O), BQ0210FS_PD_3X2_7LM_PZ_3P3 (I/O), BQ0210FS_PD_3X2_7LM_PU_3P3 (I/O), BQ0210FS_PD_3X2_7LM_PD_3P3 (I/O), BQ0210FS_PD_3X2_V2_7LM_PZ_3P3 (I/O), BQ0210FS_PD_3X2_V2_7LM_PU_3P3 (I/O), BQ0210FS_PD_3X2_V2_7LM_PD_3P3 (I/O), BQ0210FS_PU_3X2_7LM_PZ_3P3 (I/O), BQ0210FS_PU_3X2_7LM_PU_3P3 (I/O), BQ0210FS_PU_3X2_7LM_PD_3P3 (I/O), BQ0210FS_PU_3X2_V2_7LM_PZ_3P3 (I/O), BQ0210FS_PU_3X2_V2_7LM_PU_3P3 (I/O), BQ0210FS_PU_3X2_V2_7LM_PD_3P3 (I/O), BQ0212FS_3X2_7LM_PZ_3P3 (I/O), BQ0212FS_3X2_7LM_PU_3P3 (I/O), BQ0212FS_3X2_7LM_PD_3P3 (I/O), BQ0212FS_PD_3X2_7LM_PZ_3P3 (I/O), BQ0212FS_PD_3X2_7LM_PU_3P3 (I/O), BQ0212FS_PD_3X2_7LM_PD_3P3 (I/O), BQ0212FS_PU_3X2_7LM_PZ_3P3 (I/O), BQ0212FS_PU_3X2_7LM_PU_3P3 (I/O), BQ0212FS_PU_3X2_7LM_PD_3P3 (I/O), BQ0212FS_PU_3X2_V2_7LM_PZ_3P3 (I/O), BQ0212FS_PU_3X2_V2_7LM_PU_3P3 (I/O), BQ0212FS_PU_3X2_V2_7LM_PD_3P3 (I/O), BQ0213FS_PD_3X2_7LM_PD_3P3 (I/O), BQ0213FS_PD_3X2_7LM_PZ_3P3 (I/O), BQ0215FS_PD_3X2_7LM_PZ_3P3 (I/O), BQ0215FS_PD_3X2_7LM_PU_3P3 (I/O), BQ0215FS_PD_3X2_7LM_PD_3P3 (I/O), BQ0215FS_PD_3X2_V2_7LM_PZ_3P3 (I/O), BQ0215FS_PD_3X2_V2_7LM_PU_3P3 (I/O), BQ0215FS_PD_3X2_V2_7LM_PD_3P3 (I/O), BQ0215FS_PU_3X2_V2_7LM_PZ_3P3 (I/O), BQ0215FS_PU_3X2_V2_7LM_PU_3P3 (I/O), BQ0215FS_PU_3X2_V2_7LM_PD_3P3 (I/O), BQ0216FS_PD_3X2_7LM_PZ_3P3 (I/O), BQ0216FS_PD_3X2_7LM_PU_3P3 (I/O), BQ0216FS_PD_3X2_7LM_PD_3P3 (I/O), BQ0414FS_DL_3X2_7LM_PZ_3P3 (I/O), BQ0414FS_DL_3X2_7LM_PU_3P3 (I/O), BQ0414FS_DL_3X2_7LM_PD_3P3 (I/O), IQ0079FS_PD_3X2_7LM_3P3 (Input), IQ0079FS_PD_3X2_7LM_PU_3P3 (Input), IQ0079FS_PD_3X2_7LM_PD_3P3 (Input), IQ0087FS_3X2_7LM_PD_3P3 (Input), IQ0087FS_3X2_7LM_3P3 (Input), IQ0088FS_PD_3X2_7LM_3P3 (Input), IQ0088FS_PD_3X2_7LM_PU_3P3 (Input), IQ0088FS_PD_3X2_7LM_PD_3P3 (Input), IQ0088FS_PU_3X2_7LM_3P3 (Input), IQ0088FS_PU_3X2_7LM_PU_3P3 (Input), IQ0088FS_PU_3X2_7LM_PD_3P3 (Input)
